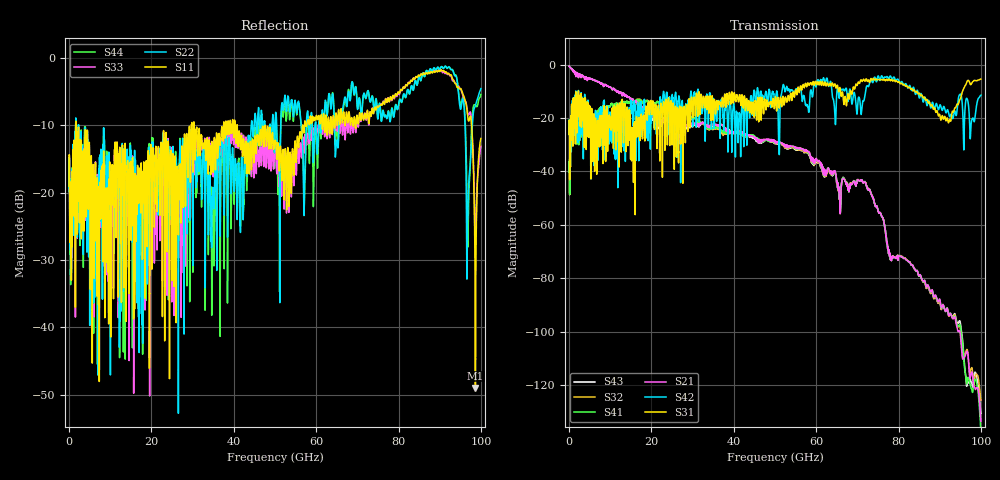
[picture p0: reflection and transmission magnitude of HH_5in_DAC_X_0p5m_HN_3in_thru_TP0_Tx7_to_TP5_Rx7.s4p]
# GHz S RI R 45
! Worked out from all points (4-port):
!   4000 points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, 25 MHz to 100 GHz, reference 45 ohm
!   strongest paths, dB at 25 MHz, 25.02 GHz, 50.02 GHz, 75.03 GHz, 100 GHz:
!     S31: -26.1, -29.2, -12.9, -5.6, -5.4
!     S42: -26.1, -11.5, -14.7, -4.3, -11.5
!     S21: -0.6, -22.0, -28.6, -54.9, -133.5
!     S41: -40.3, -16.6, -28.7, -54.9, -140.6
!     S32: -40.3, -16.6, -28.9, -54.9, -125.7
!     S43: -0.6, -22.1, -29.0, -54.9, -130.6
!   lowest |S11| = -49.0 dB at 98.67 GHz (marker M1), VSWR 1.01, Z = 45.3 + j0.00881 ohm
!   |S11| at or under -10 dB: 1.678 GHz to 29.69 GHz (28.01 GHz wide, 179 % of centre); 30.4 GHz to 37.54 GHz (7.142 GHz wide, 21 % of centre); 47.62 GHz to 56.75 GHz (9.14 GHz wide, 17.5 % of centre)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
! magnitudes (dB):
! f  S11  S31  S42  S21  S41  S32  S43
! 25 MHz  -19.0  -26.1  -26.1  -0.6  -40.3  -40.3  -0.6
! 26.57 GHz  -24.1  -32.5  -13.5  -27.4  -16.1  -16.2  -28.9
! 71.55 GHz  -9.2  -5.5  -13.6  -44.1  -44.0  -44.1  -44.0
! 90.65 GHz  -1.9  -19.1  -17.1  -90.3  -90.4  -90.2  -90.3
! 96.88 GHz  -9.1  -5.9  -14.0  -108.9  -117.1  -108.5  -118.8
! 98.67 GHz  -49.0  -6.0  -18.4  -121.7  -117.8  -116.4  -115.3
! 100 GHz  -12.0  -5.4  -11.5  -133.5  -140.6  -125.7  -130.6
